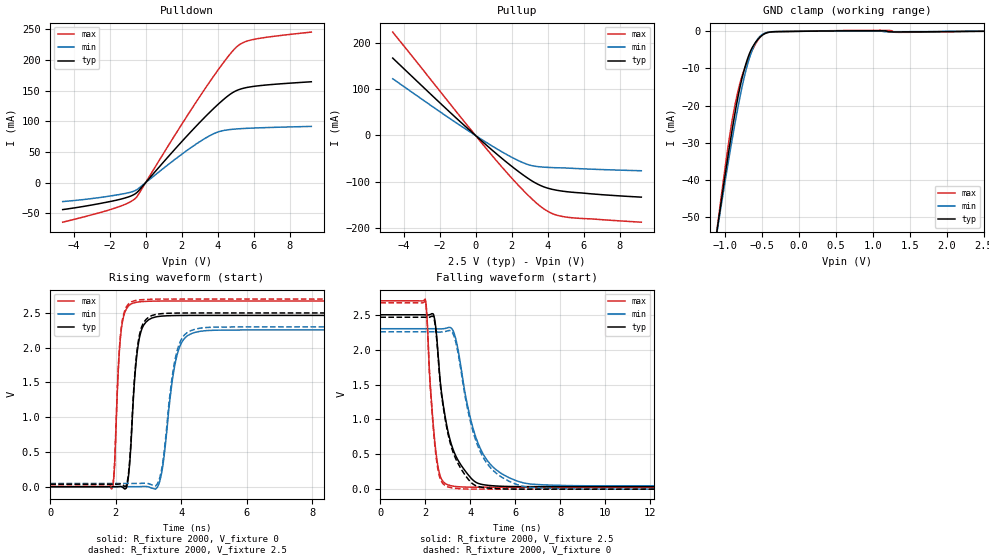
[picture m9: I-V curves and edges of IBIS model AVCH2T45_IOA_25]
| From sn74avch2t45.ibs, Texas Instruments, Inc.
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[Model]   AVCH2T45_IOA_25
Model_type  I/O
Vinl=0.7
Vinh=1.6
Enable   Active-Low
Vref =   0
Rref =   2000
Cref =   15p
Vmeas =   1.25
| variable   typ   min   max
C_comp   5.05pF   4.26pF   5.75pF
| C_pullup   4.25pF   3.21pF   5.63pF
| C_pulldown   4.37pF   3.83pF   4.80pF
| C_tri-state   5.05pF   4.26pF   5.75pF
[Temperature Range]   40   100   -40
| Ambient temperature   25   85   -40
[Voltage range]   2.5   2.3   2.7
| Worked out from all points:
|   slope of the pulldown table from 0 to 0.375 V, typ, clamps not added: 29.4 ohm
|   slope of the pullup table from 0 to 0.375 V, typ, clamps not added: 28.8 ohm
|   GND clamp passes 1 mA (typ) near -0.49 V on its own axis
|   rising waveform, R_fixture 2000, V_fixture 0: 20-80 % time 216ps typ, 349ps min, 158ps max; typ from 0 V to 2.46 V
|   falling waveform, R_fixture 2000, V_fixture 2.5: 20-80 % time 733ps typ, 1.05ns min, 341ps max; typ from 2.5 V to 0.036 V
|   rising waveform, R_fixture 2000, V_fixture 2.5: 20-80 % time 214ps typ, 345ps min, 157ps max; typ from 0.036 V to 2.5 V
|   falling waveform, R_fixture 2000, V_fixture 0: 20-80 % time 727ps typ, 1.05ns min, 333ps max; typ from 2.46 V to 0 V
[GND Clamp]
| AVCH2T45_IOA_25
|   Voltage   I(typ)   I(min)   I(max)
-4.6V     -599.7mA   -548.2mA   -664.8mA
-1.105V   -53.1mA    -53.46mA   -52.72mA
-1.08V    -49.64mA   -50.32mA   -48.82mA
-930mV    -29.72mA   -32.1mA    -27.1mA
-880mV    -23.65mA   -26.37mA   -21.29mA
-825mV    -17.62mA   -20.4mA    -16.07mA
-750mV    -11.02mA   -13.17mA   -10.85mA
-665mV    -5.769mA   -6.898mA   -6.554mA
-590mV    -3.043mA   -3.142mA   -3.475mA
-510mV    -1.266mA   -1.045mA   -1.273mA
-305mV    -86.62uA   -60.85uA   -133.1uA
2.5V      1.213nA    2.547uA    -2.967uA
[Pulldown]
| AVCH2T45_IOA_25
|   Voltage   I(typ)   I(min)   I(max)
-4.6V     -43.76mA   -30.71mA   -64.27mA
-1.715V   -29.08mA   -20.46mA   -41.45mA
-985mV    -23.44mA   -16.53mA   -33.24mA
-545mV    -17.41mA   -12.35mA   -24.86mA
1.85V     61.76mA    42.85mA    87.78mA
3.295V    106.9mA    72.08mA    152.8mA
4.12V     130.1mA    83.49mA    187.5mA
4.755V    145.2mA    86.77mA    211.8mA
5.15V     151.2mA    87.75mA    223.4mA
5.545V    154.6mA    88.42mA    229.7mA
6.15V     157.4mA    89.19mA    234.2mA
9.2V      164.4mA    91.67mA    245.2mA
[Pullup]
| AVCH2T45_IOA_25
|   Voltage   I(typ)   I(min)   I(max)
-4.6V     167.2mA    122.6mA    223.3mA
-1.155V   40.55mA    29.45mA    55.44mA
1.195V    -40.71mA   -29.18mA   -56.05mA
2.025V    -67.14mA   -47.36mA   -92.77mA
2.695V    -86.73mA   -59.71mA   -120.4mA
3.12V     -97.9mA    -65.07mA   -136.7mA
3.615V    -108.1mA   -67.81mA   -153.5mA
4.245V    -116.2mA   -69.29mA   -168.4mA
4.95V     -120.8mA   -70.1mA    -175.7mA
9.2V      -133.1mA   -76.13mA   -187.2mA
[Ramp]
| AVCH2T45_IOA_25
| variable   typ   min   max
dV/dt_r   1.50/2.21E-10   1.38/3.60E-10   1.62/1.63E-10
dV/dt_f   1.49/7.35E-10   1.36/1.05E-09   1.62/3.42E-10
R_load = 2000
[Rising Waveform]
| AVCH2T45_IOA_25
R_fixture =   2000
C_fixture =   0
L_fixture =   0
V_fixture =   0
V_fixture_min = 0
V_fixture_max = 0
|   Time   V(typ)   V(min)   V(max)
0s        27.64nV    106.2nV    1.086nV
1.895ns   31.26uV    -1.275uV   -18.99mV
1.96ns    -128.6uV   -8.971uV   280.6mV
2.175ns   28.73uV    -22.69uV   2.285V
2.385ns   138.9mV    35.5uV     2.599V
2.66ns    1.959V     -118.7uV   2.656V
3.31ns    2.45V      30.58mV    2.671V
3.88ns    2.463V     1.911V     2.672V
4.585ns   2.465V     2.237V     2.672V
34.99ns   2.465V     2.256V     2.672V
[Falling Waveform]
| AVCH2T45_IOA_25
R_fixture =   2000
C_fixture =   0
L_fixture =   0
V_fixture =   2.5
V_fixture_min = 2.3
V_fixture_max = 2.7
|   Time   V(typ)   V(min)   V(max)
0s        2.5V       2.3V       2.7V
1.995ns   2.499V     2.3V       2.722V
2.06ns    2.498V     2.3V       2.55V
2.355ns   2.512V     2.3V       919.7mV
2.505ns   2.189V     2.298V     447.8mV
2.72ns    1.386V     2.298V     143.7mV
3.135ns   667.7mV    2.314V     50.06mV
4.455ns   72.59mV    575.6mV    27.78mV
6.385ns   36.39mV    87.69mV    27.4mV
34.99ns   35.81mV    46.58mV    27.39mV
[Rising Waveform]
| AVCH2T45_IOA_25
R_fixture =   2000
C_fixture =   0
L_fixture =   0
V_fixture =   2.5
V_fixture_min = 2.3
V_fixture_max = 2.7
|   Time   V(typ)   V(min)   V(max)
0s        35.81mV    46.58mV    27.38mV
1.895ns   35.84mV    46.58mV    8.434mV
1.955ns   35.7mV     46.58mV    267.7mV
2.175ns   35.82mV    46.56mV    2.316V
2.385ns   176.1mV    46.62mV    2.627V
2.655ns   1.984V     46.44mV    2.684V
3.31ns    2.485V     78.81mV    2.699V
3.875ns   2.498V     1.961V     2.7V
4.58ns    2.5V       2.282V     2.7V
34.99ns   2.5V       2.3V       2.7V
[Falling Waveform]
| AVCH2T45_IOA_25
R_fixture =   2000
C_fixture =   0
L_fixture =   0
V_fixture =   0
V_fixture_min = 0
V_fixture_max = 0
|   Time   V(typ)   V(min)   V(max)
0s        2.465V     2.256V     2.672V
1.995ns   2.464V     2.256V     2.695V
2.065ns   2.463V     2.256V     2.498V
2.355ns   2.477V     2.256V     876.9mV
2.5ns     2.171V     2.254V     411mV
2.715ns   1.367V     2.254V     112.1mV
3.11ns    659.5mV    2.272V     23.2mV
4.44ns    31.77mV    539.2mV    382.7uV
6.34ns    510.9uV    40.79mV    14.7uV
34.99ns   703.2nV    336.5nV    366.8nV
